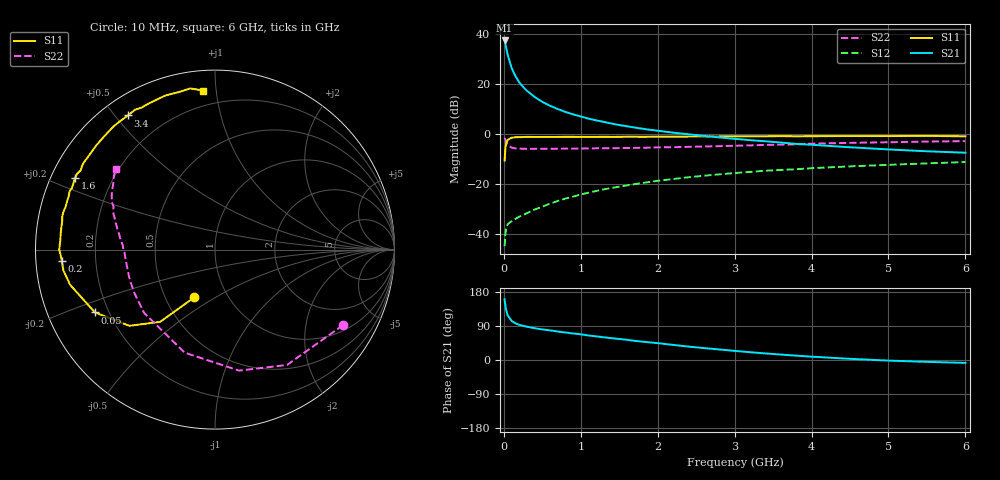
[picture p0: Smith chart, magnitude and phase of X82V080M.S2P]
! SIEMENS Small Signal Semiconductors
! BFP136W
! Si NPN RF Bipolar Junction Transistor in SOT343
! VCE = 2 V  IC = 80 mA
! Common Emitter S-Parameters:  September  1994
# GHz  S  MA  R  50
!  f  S11  S21  S12  S22
! GHz  MAG  ANG  MAG  ANG  MAG  ANG  MAG  ANG
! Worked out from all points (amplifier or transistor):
!   40 points, 10 MHz to 6 GHz, reference 50 ohm
!   highest |S21| = 37.4 dB at 10 MHz (marker M1)
!   |S21| within 3 dB of that: start of sweep to 31.31 MHz
!   unconditionally stable (mu >= 1): 493.5 MHz to 2.891 GHz
!   at 200 MHz: K = 0.67, MSG = 26.9 dB, |S12| = -33.2 dB
!   at 1.5 GHz: K = 1.11, MAG = 10.3 dB, |S12| = -21.2 dB
!   at 6 GHz: K = 0.98, MSG = 1.9 dB, |S12| = -11.3 dB
!   S11 on the Smith chart (normalised r, x): 10 MHz: 0.70, -0.40; 50 MHz: 0.15, -0.24; 200 MHz: 0.08, -0.04; 1.6 GHz: 0.07, +0.24; 3.4 GHz: 0.07, +0.54; 6 GHz: 0.11, +0.92
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0.01  0.2903 -113.5  74.17 160.2  0.0056 68.2  0.8284 -30.5
0.02  0.5053 -127.2  63.73 143.7  0.0098 57.2  0.7577 -58.0
0.03  0.6384 -138.3  53.69 132.0  0.0123 48.4  0.6876 -78.7
0.05  0.7551 -152.4  38.24 117.9  0.0154 38.6  0.5986 -106.4
0.1  0.8311 -166.4  21.12 103.3  0.0177 34.6  0.5296 -138.2
0.15  0.8529 -172.3  14.37 96.8  0.0197 37.3  0.5103 -151.5
0.2  0.8558 -175.6  10.78 92.9  0.0219 40.4  0.5042 -158.6
0.25  0.8615 -178.3  8.691 90.0  0.0235 44.0  0.502 -163.1
0.3  0.868 -179.9  7.266 87.9  0.0257 46.7  0.4997 -166.1
0.4  0.8634 176.5  5.472 83.9  0.0303 51.4  0.4998 -170.2
0.5  0.8645 173.9  4.365 80.7  0.0347 54.9  0.5004 -172.9
0.6  0.8648 171.9  3.638 78.2  0.0397 57.1  0.5013 -174.7
0.7  0.866 169.4  3.139 75.1  0.0451 59.3  0.5026 -176.0
0.8  0.8708 167.8  2.744 72.6  0.0503 59.9  0.5038 -177.3
1.1  0.867 161.6  2.013 64.6  0.066 61.3  0.5091 179.9
1.6  0.8757 153.0  1.413 53.3  0.0925 60.0  0.5199 176.0
2.2  0.8761 142.8  1.054 39.9  0.1241 55.7  0.5384 171.4
3.2  0.8898 125.9  0.746 20.6  0.1721 46.0  0.5855 162.6
3.4  0.891 123.0  0.708 17.3  0.1818 43.9  0.5991 160.7
4.5  0.9019 107.8  0.537 3.1  0.2224 33.5  0.6585 150.8
5.5  0.9085 98.7  0.446 -4.9  0.2554 25.5  0.698 143.8
6  0.8889 94.3  0.418 -7.6  0.2717 21.1  0.7133 140.8
